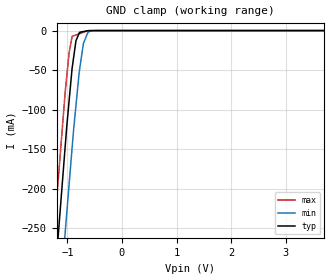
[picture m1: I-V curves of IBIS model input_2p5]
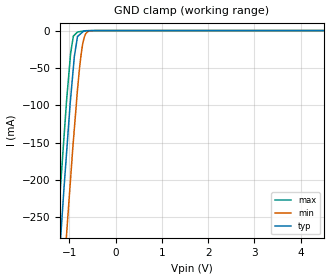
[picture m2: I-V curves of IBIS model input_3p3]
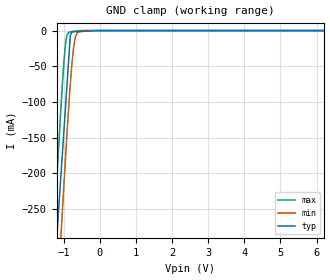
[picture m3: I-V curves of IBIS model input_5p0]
| Texas Instruments Incorporated
| ADS8167 8-Channel, 16-Bit, 1-MSPS SAR ADC With Easy to Drive Analog Inputs
| Marketing part#   Digital Voltage Range   Package-type   #pins
| ADS8167   2.35V - 5.5V   VQFN   32
[IBIS Ver]   4.1
[File name]   ads8167.ibs
[File Rev]   1.0
[Date]   08/08/2017
[Source]
| Texas Instruments Incorporated.
| Analog-eLab Design Center, HPA
| 12500 TI Blvd
| Dallas, TX -75243
[Notes]   Revision History:
| Rev 1.0: 08/08/2017
| - Initial version of the model
| - Model generated from simulations in SPECTRE
| - Model matched to SPICE simulation
| - C_comp although listed in numerical order of value are
|   obtained from varying PVT conditions. For PVT conditions for
|   each specific value refer the buffer description under
|   respective [Model]. IBIS model user is responsible for using
|   appropriate C_comp to simulate for Signal Integrity.
| - Warnings regarding combined Non-monotonicity of various models have been
|   reviewed and considered minor and can be ignored.
[Disclaimer]
| This model is designed as an aid for customers of Texas Instruments.
| TI and its licensors and suppliers make no warranties, either expressed
| or implied, with respect to this  model, including the warranties of
| merchantability or fitness for a particular purpose. The model is
| provided solely on an "as is" basis. The entire risk as to its quality
| and performance is with the customer.
[Copyright]
(C) Copyright 2017 Texas Instruments Incorporated.All rights reserved.
|   ADS8167
[Component]   ADS8167
[Manufacturer]   TI
[Package]   |32 VQFN
|   typ   min   max
R_pkg   0.1   0.08   0.12
L_pkg   1.0nH   0.8nH   1.2nH
C_pkg   0.2pF   0.16pF   0.24pF
[Pin] signal_name  model_name   R_pin   L_pin   C_pin
1   AGND   power   NA   NA   NA
2   DECAP   power   NA   NA   NA
3   REFIO   nc   NA   NA   NA
4   REFM   nc   NA   NA   NA
5   REFP   nc   NA   NA   NA
6   REFP   nc   NA   NA   NA
7   REF/2   nc   NA   NA   NA
8   AIN-COM   nc   NA   NA   NA
9   AIN0   nc   NA   NA   NA
10   AIN1   nc   NA   NA   NA
11   AIN2   nc   NA   NA   NA
12   AIN3   nc   NA   NA   NA
13   AIN4   nc   NA   NA   NA
14   AIN5   nc   NA   NA   NA
15   AIN6   nc   NA   NA   NA
16   AIN7   nc   NA   NA   NA
17   ADC-AINP   nc   NA   NA   NA
18   MUXOUT-P   nc   NA   NA   NA
19   MUXOUT-M   nc   NA   NA   NA
20   ADC-AINM   nc   NA   NA   NA
21   AGND   power   NA   NA   NA
22   ALARM   tri_state   NA   NA   NA
23   CSz   input   NA   NA   NA
24   SDI   input   NA   NA   NA
25   SCLK   input   NA   NA   NA
26   SDO-0   tri_state   NA   NA   NA
27   SDO-1/SEQ_ACTIVE  tri_state   NA   NA   NA
28   RVS   tri_state   NA   NA   NA
29   RSTz   input   NA   NA   NA
30   DVDD   power   NA   NA   NA
31   DGND   power   NA   NA   NA
32   AVDD   power   NA   NA   NA
|   Model Selectors
[Model Selector] tri_state
tri_state_2p5   2.5V  digital 3-state
tri_state_3p3   3.3V  digital 3-state
tri_state_5p0   5.0V  digital 3-state
[Model Selector] input
input_2p5   2.5V  digital input
input_3p3   3.3V  digital input
input_5p0   5.0V  digital input
| Models and submodels in the file (6): input_2p5 (Input), input_3p3 (Input), input_5p0 (Input), tri_state_2p5 (3-state), tri_state_3p3 (3-state), tri_state_5p0 (3-state)
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|   input_2p5 Model
[Model]   input_2p5
Model_type   Input
Vinl = 0.75
Vinh = 1.75
|   typ   min   max
C_comp   3.6788E-13F  3.5370E-13F  3.8163E-13F
|  Where Nom  PVT is Nominal Process, 2.5V,   27C
|   Fast PVT is Strong Process,  2.65V,  -40C
|   Slow PVT is Weak Process,   2.35V, 125C
[Model spec]
|subparameter
Vinl   0.75   0.705   0.795
Vinh   1.75   1.645   1.855
[Voltage Range]   2.5   2.35   2.65
|Junction Temperature
[Temperature Range]   27   125   -40
[Power Clamp Reference]   2.5   2.35   2.65
[GND Clamp Reference]   0   0   0
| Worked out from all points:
|   GND clamp passes 1 mA (typ) near -0.69 V on its own axis
[GND Clamp]
|   Voltage   I(typ)   I(min)   I(max)
-2.5V     -1.542A    -1.65A     -1.476A
-1.257V   -339.3mA   -450.7mA   -268.7mA
-1.2V     -286.1mA   -399.3mA   -215.5mA
-1.041V   -146.3mA   -255.1mA   -77.71mA
-969.2mV  -88.7mA    -194.2mA   -27.95mA
-913.7mV  -47.32mA   -147.6mA   -7.24mA
-843.8mV  -12.85mA   -94.75mA   -5.542mA
-778.6mV  -2.234mA   -49.86mA   -3.955mA
-706.6mV  -1.238mA   -16.12mA   -2.204mA
-624.9mV  -108.2uA   -2.432mA   -218.2uA
-543.2mV  -22.37uA   -316.5uA   -42.63uA
5V        0A         0A         0A
[POWER Clamp]
|   Voltage   I(typ)   I(min)   I(max)
-2.5V     0A         0A         0A
0V        0A         0A         0A
5V        0A         0A         0A
|   input_3p3 Model
[Model]   input_3p3
Model_type   Input
Vinl = 0.99
Vinh = 2.31
|   typ   min   max
C_comp   3.5579E-13F  3.4345E-13F  3.6914E-13F
|  Where Nom  PVT is Nominal Process, 3.3V,   27C
|   Fast PVT is Strong Process,  3.6V,   -40C
|   Slow PVT is Weak Process,   3.0V,   125C
[Model spec]
|subparameter
Vinl   0.99   0.9   1.08
Vinh   2.31   2.1   2.52
[Voltage Range]   3.3   3   3.6
|Junction Temperature
[Temperature Range]   27   125   -40
[Power Clamp Reference]   3.3   3   3.6
[GND Clamp Reference]   0   0   0
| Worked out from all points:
|   GND clamp passes 1 mA (typ) near -0.70 V on its own axis
[GND Clamp]
|   Voltage   I(typ)   I(min)   I(max)
-3.3V     -2.332A    -2.436A    -2.268A
-1.26V    -342.5mA   -453.9mA   -271.8mA
-1.206V   -293.1mA   -404.9mA   -221.2mA
-1.12V    -213.9mA   -326.3mA   -145.6mA
-1.063V   -164.9mA   -274.1mA   -94.94mA
-973.4mV  -90.66mA   -197.2mA   -30.29mA
-914.6mV  -49.66mA   -147.9mA   -7.415mA
-825mV    -7.92mA    -79.1mA    -1.904mA
-705.4mV  -1.538mA   -15.75mA   -741.1uA
-650.7mV  -211.1uA   -4.628mA   -389.3uA
-540mV    -51.86uA   -293.1uA   -98.9uA
6.6V      0A         0A         0A
[POWER Clamp]
|   Voltage   I(typ)   I(min)   I(max)
-3.3V     0A         0A         0A
0V        0A         0A         0A
6.6V      0A         0A         0A
|   input_5p0 Model
[Model]   input_5p0
Model_type   Input
Vinl = 1.5
Vinh = 3.5
|   typ   min   max
C_comp   3.3685E-13F  3.2537E-13F  3.4812E-13F
|  Where Nom  PVT is Nominal Process, 5V,   27C
|   Fast PVT is Strong Process,  5.5V, -40C
|   Slow PVT is Weak Process,   4.5V, 125C
[Model spec]
|subparameter
Vinl   1.5   1.35   1.65
Vinh   3.5   3.15   3.75
[Voltage Range]   5   4.5   5.5
|Junction Temperature
[Temperature Range]   27   125   -40
[Power Clamp Reference]   5   4.5   5.5
[GND Clamp Reference]   0   0   0
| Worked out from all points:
|   GND clamp passes 1 mA (typ) near -0.43 V on its own axis
[GND Clamp]
|   Voltage   I(typ)   I(min)   I(max)
-5V       -4.018A    -4.118A    -3.957A
-1.43V    -502.2mA   -614.3mA   -431.8mA
-1.25V    -331.9mA   -444.3mA   -261.2mA
-1.094V   -214.5mA   -302mA     -121.1mA
-1.039V   -173.3mA   -253.6mA   -76.09mA
-962.4mV  -115.5mA   -187.5mA   -24.33mA
-903.8mV  -71.28mA   -138.6mA   -5.665mA
-818mV    -6.614mA   -74.89mA   -1.804mA
-724.2mV  -1.671mA   -22.3mA    -1.081mA
-677.8mV  -1.564mA   -8.785mA   -724.7uA
-415.9mV  -959.8uA   -12.38uA   -3.418uA
10V       0A         0A         0A
[POWER Clamp]
|   Voltage   I(typ)   I(min)   I(max)
-5V       0A         0A         0A
0V        0A         0A         0A
10V       0A         0A         0A
